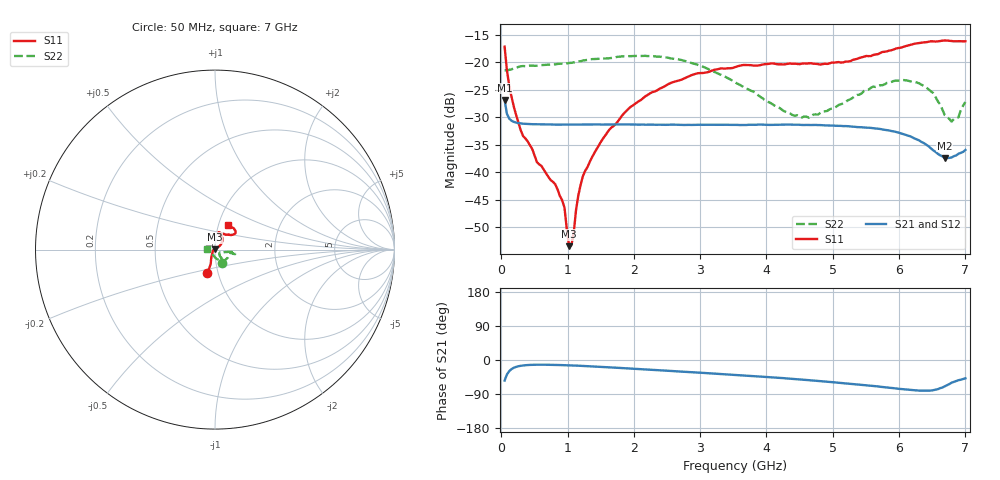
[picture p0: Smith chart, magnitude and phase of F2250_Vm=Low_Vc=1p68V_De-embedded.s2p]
! Integrated Device Technology
! Corporate Headquarters
! 6024 Silver Creek Valley Road
! San Jose, CA 95138  USA
! Phone:  1-408-284-8200
! Toll Free:  1-800-223-1366
! Webpage:  http://www.idt.com/
! Timing and RF Division
! 515 Groton Road, Suite 102
! Westford, MA 01886-6024
! Device:  F2250
! Description: Voltage Variable RF Attenuator
! Frequency:  50.0 -  6000.00 MHz
! Package:  3x3 mm Thin QFN Plastic Package: 16 pin
! Ports:  2 RF, 3 DC
!  Pin  1  = GND
!  Pin  2  = NC
!  Pin  3  = RF1  = Port 1
!  Pin  4  = NC
!  Pin  5  = GND
!  Pin  6  = GND
!  Pin  7  = GND
!  Pin  8  = GND
!  Pin  9  = NC
!  Pin 10  = RF2  = Port 2
!  Pin 11  = NC
!  Pin 12  = GND
!  Pin 13  = GND
!  Pin 14  = VCNTRL
!  Pin 15  = VDD
!  Pin 16  = VMODE
! Vcntrl:  1.680 Volts
! Vmode:  +0.000 Volts
! Vdd:  +3.30  Volts
! Current:  1.189 mA
! Data:  The device was measured on a the F2250 evaluation board which has
!  individual transmission lines to the RF pins.  Data was collected
!  using a calibrated network analyzer.  The evaluation board was
!  de-embedded using a TRL calibration technique.
!  The reference plane is the edge of the package pin.
! Misc:  SN 10
!  Action Tracker AT0258
! Date Measured:  2014-11-26
! Date:  2015-10-15  MJV
! Note:
!  Integrated Device Technology supplies this data as a sample of measured
!  data at the package pin for this product.  Your particular data for this
!  product may vary.
!  Data was taken at 25 degrees C.
!  Integrated Device Technology reserves the right to change this data at anytime.
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# GHz S dB R 50
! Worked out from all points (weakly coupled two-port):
!   201 points, 50 MHz to 7 GHz, reference 50 ohm
!   highest |S21| = -26.86 dB at 50 MHz (marker M1); lowest = -37.4 dB at 6.687 GHz (marker M2)
!   lowest |S11| = -53.4 dB at 1.023 GHz (marker M3), VSWR 1.00, Z = 49.8 + j0.146 ohm
!   |S11| at or under -10 dB: start of sweep to end of sweep
!   |S22| runs from -30.8 to -18.8 dB; largest |S21 - S12| = 9e-05
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0.05  -17.15 -107.9  -26.86 -54.2  -26.86 -54.2  -21.47 -63.8
0.1195  -24.20 -110.7  -30.23 -29.3  -30.23 -29.3  -21.37 -20.1
0.29325  -32.35 -125.3  -31.11 -15.3  -31.12 -15.3  -20.72 -10.3
0.91875  -45.09 157.5  -31.31 -13.5  -31.32 -13.5  -20.23 -11.7
0.9535  -46.44 171.6  -31.31 -13.7  -31.33 -13.7  -20.33 -11.6
1.023  -53.43 136.5  -31.30 -14.1  -31.32 -14.1  -20.11 -11.4
1.05775  -53.28 105.7  -31.31 -14.3  -31.34 -14.3  -20.09 -11.4
1.162  -44.19 46.6  -31.32 -15.0  -31.32 -15.0  -19.83 -12.7
1.2315  -40.66 38.1  -31.31 -15.6  -31.31 -15.6  -19.67 -13.3
1.6485  -31.99 39.6  -31.31 -19.5  -31.31 -19.5  -19.23 -12.9
1.9265  -28.34 39.9  -31.31 -22.4  -31.32 -22.4  -18.87 -12.6
2.37825  -24.87 46.3  -31.34 -27.0  -31.36 -27.0  -18.95 -11.0
3.525  -20.87 72.0  -31.37 -39.4  -31.39 -39.4  -23.63 -12.2
4.39375  -20.25 76.6  -31.34 -49.9  -31.33 -49.9  -29.59 -29.0
4.7065  -20.25 72.1  -31.38 -54.2  -31.38 -54.2  -29.49 -41.2
5.85325  -17.86 40.1  -32.40 -73.2  -32.40 -73.2  -23.65 -57.3
6.3745  -16.36 41.1  -34.69 -81.0  -34.67 -81.1  -24.29 -69.6
6.5135  -16.18 44.2  -35.99 -79.7  -35.97 -79.7  -25.58 -80.2
6.68725  -16.02 48.5  -37.39 -69.6  -37.38 -69.5  -29.57 -106.0
6.7915  -16.13 52.0  -37.31 -59.9  -37.29 -59.9  -30.78 -135.0
6.89575  -16.13 56.8  -36.63 -53.3  -36.64 -53.1  -30.00 -163.8
7  -16.17 63.0  -35.93 -48.3  -35.93 -48.3  -27.21 175.7
